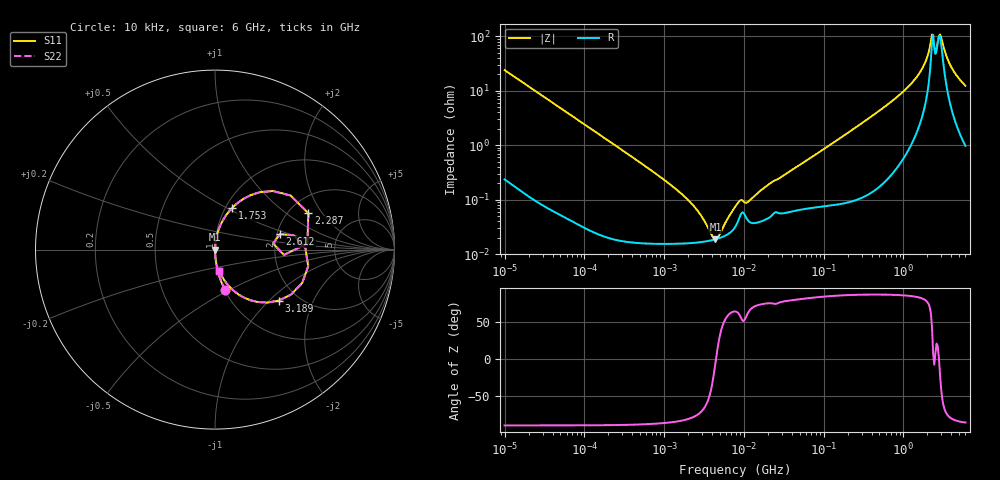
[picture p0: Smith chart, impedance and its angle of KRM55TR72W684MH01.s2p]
!Murata Part Number: KRM55TR72W684MH01
!These Parameters are Measured in Series Mode Connection
!Data Generated on Jan 08, 2026
!  o--ll--o
!Port1  Port2
!  o------o
!Operation Temp=25[degC], DC Bias Voltage=0[V]
!Freq. Start=10[kHz] Stop=6[GHz] 401[Steps]
# Hz S RI R 50
!Freq.(Hz) S11(Real) S11(Imag) S21(Real) S21(Imag) S12(Real) S12(Imag) S22(Real) S22(Imag)
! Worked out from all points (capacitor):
!   401 points, 10 kHz to 6 GHz, reference 50 ohm
!   read as one part in series: C = 665 nF near 10.69 kHz
!   lowest |Z| = 18.7 mohm at 4.401 MHz (marker M1)
!   series resonance near 4.47 MHz, so ESL is about 1.9 nH
!   S11 on the Smith chart (normalised r, x): 10 kHz: 1.00, -0.48; 1.753 GHz: 1.07, +0.53; 2.287 GHz: 2.54, +1.50; 2.612 GHz: 2.08, +0.42; 3.189 GHz: 1.60, -1.14; 6 GHz: 1.02, -0.24
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10000  0.056 -0.225  0.944 0.225  0.944 0.225  0.056 -0.225
26237  0.00917 -0.0906  0.9908 0.0906  0.9908 0.0906  0.00917 -0.0906
92862  0.000997 -0.026  0.999 0.026  0.999 0.026  0.000997 -0.026
862344  0.000161 -0.00271  0.9998 0.00271  0.9998 0.00271  0.000161 -0.00271
2262542  0.00016 -0.000798  0.9998 0.000798  0.9998 0.000798  0.00016 -0.000798
4400522  0.000187 -1.69e-05  0.9998 1.69e-05  0.9998 1.69e-05  0.000187 -1.69e-05
4862284  0.000195 9.25e-05  0.9998 -9.25e-05  0.9998 -9.25e-05  0.000195 9.25e-05
7745967  0.000311 0.000663  0.9997 -0.000663  0.9997 -0.000663  0.000311 0.000663
9147502  0.000535 0.00082  0.9995 -0.00082  0.9995 -0.00082  0.000535 0.00082
1.15457e7  0.0004 0.000846  0.9996 -0.000846  0.9996 -0.000846  0.0004 0.000846
2.172113e7  0.000494 0.00196  0.9995 -0.00196  0.9995 -0.00196  0.000494 0.00196
7.193098e7  0.000741 0.00606  0.9993 -0.00606  0.9993 -0.00606  0.000741 0.00606
6.67969e8  0.00602 0.0585  0.994 -0.0585  0.994 -0.0585  0.00602 0.0585
1.215551e9  0.0248 0.1235  0.9752 -0.1235  0.9752 -0.1235  0.0248 0.1235
1.752557e9  0.0942 0.2308  0.9058 -0.2308  0.9058 -0.2308  0.0942 0.2308
2.069661e9  0.251 0.3202  0.749 -0.3202  0.749 -0.3202  0.251 0.3202
2.286837e9  0.5202 0.2029  0.4798 -0.2029  0.4798 -0.2029  0.5202 0.2029
2.612262e9  0.363 0.0873  0.637 -0.0873  0.637 -0.0873  0.363 0.0873
2.886376e9  0.5191 -0.0933  0.4809 0.0933  0.4809 0.0933  0.5191 -0.0933
3.189254e9  0.3547 -0.2842  0.6453 0.2842  0.6453 0.2842  0.3547 -0.2842
4.025378e9  0.0999 -0.2258  0.9001 0.2258  0.9001 0.2258  0.0999 -0.2258
6e9  0.024 -0.1184  0.976 0.1184  0.976 0.1184  0.024 -0.1184
